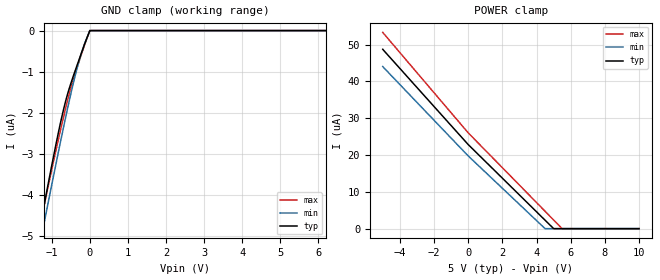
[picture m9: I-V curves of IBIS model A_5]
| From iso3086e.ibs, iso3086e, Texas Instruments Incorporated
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|   A_5 Model
[Model]   A_5
Model_type   Input
|Signals   A   positive pin
|Rref = 27   Note: 54 Ohm differential load;
Vinl   = 0.8
Vinh   = 2
| C_comp   obtained at 20MHz
|   typ   min   max
C_comp   5.334fF   5.274f   5.390fF
[Voltage Range]   5   4.5   5.5
[Temperature Range]   40   125   -40
[Power Clamp Reference]   5   4.5   5.5
[GND Clamp Reference]   0   0   0
[GND Clamp]
|   Voltage   I(typ)   I(min)   I(max)
-5V       -23.77uA   -23.05uA   -24.37uA
-1.377V   -5.139uA   -5.531uA   -5.071uA
-1.272V   -4.618uA   -5.036uA   -4.595uA
-1.235V   -4.433uA   -4.86uA    -4.428uA
-875mV    -2.716uA   -3.193uA   -2.868uA
-747.5mV  -2.161uA   -2.618uA   -2.343uA
-642.5mV  -1.753uA   -2.156uA   -1.929uA
-470mV    -1.214uA   -1.435uA   -1.313uA
-305mV    -773.3nA   -826.1nA   -818.5nA
-132.5mV  -322.2nA   -315.3nA   -341nA
2.5mV     0A         0A         0A
10V       0A         0A         0A
[POWER Clamp]
|   Voltage   I(typ)   I(min)   I(max)
-5V       48.71uA    44.02uA    53.3uA
2.5mV     22.84uA    19.75uA    26.02uA
4.503V    2.294uA    0A         4.721uA
5.005V    0A         0A         2.343uA
5.5V      0A         0A         0A
10V       0A         0A         0A
